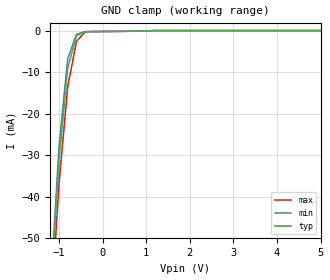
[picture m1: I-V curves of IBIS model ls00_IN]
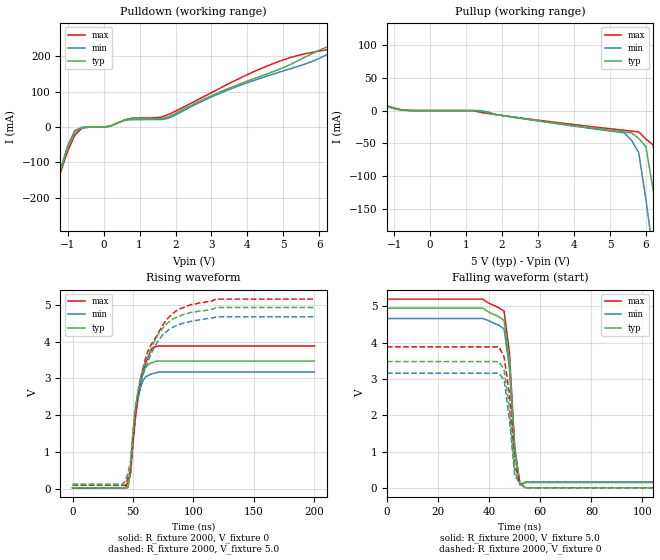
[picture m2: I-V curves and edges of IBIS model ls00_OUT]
|   TEXAS INSTRUMENTS INCORPORATED
|   Standard Linear and Logic Group
|   IBIS Model of SN74LS00
|   QUADRUPLE 2-INPUT POSITIVE-NAND GATES
|   SOIC 14-pin (D), SOP 14-pin (NS), SSOP 14-pin (DB), P-DIP 14-pin (N)
[IBIS Ver]   3.2
[Comment Char]  |_char
[File Name]   sn74ls00.ibs
[File Rev]   3.2
|[Date]   11/11/04
[Source]   File originated at Texas Instruments, Inc.
[Notes]   The following is a sample IBIS file for the LS00.
   - FILE REV HISTORY
   - 3.2 Re-Release IBIS file on 11/11/04
   - Power clamp data deleted as there is no power-clamp diode.
   - All test data contained in this file are derived from
   actual measurements.
   - The measurement used NS package.
   - File created by Nobuhisa Ohtsubo, SLL Product Engineering.
[Disclaimer] Property of Texas Instruments Incorporated.  Unauthorized
   reproduction and/or distribution is strictly prohibited.
   This product is protected under copyright law.
   Created 2000, (C) Copyright 2000, Texas Instruments Inc.,
   All Rights Reserved.
   UNLESS THERE IS A SIGNED, WRITTEN AGREEMENT TO THE
   CONTRARY, TEXAS INSTRUMENTS () IS PROVIDING THE IBIS
   MODELS  AND WITHOUT ANY WARRANTY, EXPRESSED OR
   IMPLIED.  TI assumes no liability for:
   1) the accuracy of the IBIS models provided to your
   company;
   2) the proper functioning of these IBIS Models in your
   design or for any resulting applications; or
   3) infringement of patents, copyrights or intellectual
   property rights resulting from your use of these IBIS
   models.
   TI provides IBIS Models as a service to our customers.
   You and your company shall not distribute, sell or give
   these models to anyone else without prior written
   permission from TI.
   TI reserves the right to make changes to our products or
   to discontinue any semiconductor product or service
   without notice, and advises our customers to obtain the
   latest version of relevant information to verify, before
   placing orders, that the information being relied on is
   current.
   Please be aware that your receipt and use of the IBIS
   information provided shall serve as acceptance of these
   terms and conditions.  If you do not accept these terms,
   you should return or destroy the IBIS models and any
   other accompanying information immediately.
|   Component ls00_D
[Component]   ls00_D
[Manufacturer]  Texas Instruments, Inc.
[Package]
|   typ   min   max
R_pkg   0.031   0.028   0.034
L_pkg   3.109nH   2.462nH   3.889nH
C_pkg   0.473pF   0.363pF   0.628pF
[Pin]   signal_name   model_name   R_pin   L_pin   C_pin
1   1A   ls00_IN   0.033   3.854nH   0.622pF
2   1B   ls00_IN   0.032   3.188nH   0.473pF
3   1Y   ls00_OUT   0.028   2.462nH   0.377pF
4   2A   ls00_IN   0.031   2.596nH   0.363pF
5   2B   ls00_IN   0.028   2.521nH   0.372pF
6   2Y   ls00_OUT   0.034   3.250nH   0.476pF
7   GND   GND   0.034   3.889nH   0.628pF
8   3Y   ls00_OUT   0.034   3.889nH   0.628pF
9   3A   ls00_IN   0.034   3.250nH   0.476pF
10   3B   ls00_IN   0.028   2.521nH   0.372pF
11   4Y   ls00_OUT   0.031   2.596nH   0.364pF
12   4A   ls00_IN   0.028   2.462nH   0.377pF
13   4B   ls00_IN   0.032   3.188nH   0.473pF
14   VCC   POWER   0.033   3.854nH   0.622pF
|   Component ls00_NS
[Component]   ls00_NS
[Manufacturer]  Texas Instruments, Inc.
[Package]
|   typ   min   max
R_pkg   0.045   0.039   0.054
L_pkg   3.796nH   2.561nH   4.952nH
C_pkg   0.528pF   0.288pF   0.710pF
[Pin]   signal_name   model_name   R_pin   L_pin   C_pin
1   1A   ls00_IN   0.047   4.867nH   0.706pF
2   1B   ls00_IN   0.051   4.083nH   0.592pF
3   1Y   ls00_OUT   0.041   2.915nH   0.376pF
4   2A   ls00_IN   0.039   2.561nH   0.288pF
5   2B   ls00_IN   0.041   3.101nH   0.430pF
6   2Y   ls00_OUT   0.047   4.047nH   0.589pF
7   GND   GND   0.051   4.909nH   0.700pF
8   3Y   ls00_OUT   0.045   4.784nH   0.694pF
9   3A   ls00_IN   0.054   4.176nH   0.597pF
10   3B   ls00_IN   0.039   3.287nH   0.449pF
11   4Y   ls00_OUT   0.039   2.586nH   0.294pF
12   4A   ls00_IN   0.040   2.802nH   0.371pF
13   4B   ls00_IN   0.049   4.080nH   0.593pF
14   VCC   POWER   0.052   4.952nH   0.710pF
|   Component ls00_DB
[Component]   ls00_DB
[Manufacturer]  Texas Instruments, Inc.
[Package]
|   typ   min   max
R_pkg   0.044   0.041   0.046
L_pkg   3.551nH   3.258nH   3.927nH
C_pkg   0.402pF   0.360pF   0.421pF
[Pin]   signal_name   model_name   R_pin   L_pin   C_pin
1   1A   ls00_IN   0.046   3.927nH   0.408pF
2   1B   ls00_IN   0.044   3.587nH   0.421pF
3   1Y   ls00_OUT   0.041   3.289nH   0.398pF
4   2A   ls00_IN   0.042   3.258nH   0.360pF
5   2B   ls00_IN   0.041   3.286nH   0.403pF
6   2Y   ls00_OUT   0.044   3.586nH   0.421pF
7   GND   GND   0.046   3.927nH   0.408pF
8   3Y   ls00_OUT   0.046   3.927nH   0.408pF
9   3A   ls00_IN   0.044   3.586nH   0.421pF
10   3B   ls00_IN   0.041   3.286nH   0.403pF
11   4Y   ls00_OUT   0.043   3.258nH   0.360pF
12   4A   ls00_IN   0.041   3.289nH   0.398pF
13   4B   ls00_IN   0.044   3.587nH   0.421pF
14   VCC   POWER   0.046   3.927nH   0.408pF
|   Component ls00_N
[Component]   ls00_N
[Manufacturer]   Texas Instruments, Inc.
[Package]
|   typ   min   max
R_pkg   4.500e-02   3.700e-02   6.300e-02
L_pkg   5.407e-09   3.922e-09   6.942e-09
C_pkg   3.890e-13   2.050e-13   6.040e-13
[Pin]   signal_name   model_name   R_pin   L_pin   C_pin
1   1A   ls00_IN   6.300e-02   6.942e-09   6.040e-13
2   1B   ls00_OUT   3.700e-02   6.200e-09   4.060e-13
3   1Y   ls00_IN   4.200e-02   4.389e-09   3.220e-13
4   2A   ls00_OUT   3.800e-02   3.922e-09   2.050e-13
5   2B   ls00_IN   3.900e-02   4.301e-09   2.980e-13
6   2Y   ls00_OUT   3.800e-02   5.329e-09   3.560e-13
7   GND   GND   5.300e-02   6.510e-09   5.440e-13
8   3Y   ls00_OUT   5.300e-02   6.437e-09   5.390e-13
9   3A   ls00_IN   3.900e-02   5.352e-09   3.470e-13
10   3B   ls00_OUT   4.200e-02   4.473e-09   2.970e-13
11   4Y   ls00_IN   4.400e-02   4.326e-09   2.250e-13
12   4A   ls00_OUT   4.200e-02   4.295e-09   2.800e-13
13   4B   ls00_IN   4.200e-02   6.318e-09   4.180e-13
14   VCC   POWER   6.100e-02   6.900e-09   6.030e-13
| Models and submodels in the file (2): ls00_IN (Input), ls00_OUT (Output)
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|   Model ls00_IN
[Model]   ls00_IN
Model_type  Input
Polarity   Inverting
Vinl = 0.8
Vinh = 2.0
| variable   typ   min   max
C_comp   1.33pf   1.00pf   1.66pf
[Temperature Range]   25   0   70
[Voltage Range]   5.0   4.75   5.25
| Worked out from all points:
|   GND clamp passes 1 mA (typ) near -0.55 V on its own axis
[GND Clamp]
|   Voltage   I(typ)   I(min)   I(max)
-5V       -1.018A    -1.077A    -921.2mA
-1.2V     -66.4mA    -63.52mA   -70.37mA
-1V       -31.36mA   -27.9mA    -37.06mA
-800mV    -9.019mA   -6.772mA   -13.61mA
-600mV    -1.272mA   -876.1uA   -2.626mA
-400mV    -255.9uA   -254.9uA   -323.7uA
-200mV    -235.6uA   -242.4uA   -213.5uA
1.2V      -728.9nA   -2.758uA   -68.03nA
5V        8.6nA      8.752nA    16.82nA
|   Model ls00_OUT
[Model]   ls00_OUT
Model_type  Output
Polarity   Non-Inverting
Vmeas = 1.3v
Cref = 15pf
Rref = 2000
Vref = 0V
| variable   typ   min   max
C_comp   5.8pf   4.35pf   7.25pf
[Temperature Range]   25   0   70
[Voltage Range]   5.0   4.75   5.25
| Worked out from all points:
|   slope of the pulldown table from 0 to 0.75 V, typ, clamps not added: 32.8 ohm
|   slope of the pullup table from 0 to 0.75 V, typ, clamps not added: 31.9 kohm
|   rising waveform, R_fixture 2000, V_fixture 0: 20-80 % time 7.12ns typ, 6.53ns min, 8.96ns max; typ from 0.022 V to 3.47 V
|   falling waveform, R_fixture 2000, V_fixture 5.0: 20-80 % time 2.91ns typ, 2.91ns min, 2.89ns max; typ from 4.95 V to 0.156 V
|   rising waveform, R_fixture 2000, V_fixture 5.0: 20-80 % time 18.3ns typ, 17.6ns min, 19.9ns max; typ from 0.11 V to 4.93 V
|   falling waveform, R_fixture 2000, V_fixture 0: 20-80 % time 2.93ns typ, 2.92ns min, 3.01ns max; typ from 3.48 V to 0.011 V
[Pulldown]
|   Voltage   I(typ)   I(min)   I(max)
-5V       -1.623A    -1.707A    -1.473A
-1.8V     -355.8mA   -364.5mA   -338.6mA
-1.6V     -276.6mA   -280.8mA   -267.5mA
-1.2V     -124mA     -120.4mA   -129.6mA
-1V       -58.61mA   -53.03mA   -68.64mA
-800mV    -14.32mA   -10.47mA   -22.99mA
-600mV    -1.475mA   -1.096mA   -3.152mA
1.8V      28.53mA    24.12mA    35.15mA
5V        167.6mA    158.3mA    189.4mA
6.4V      233.2mA    215.8mA    221.3mA
7.8V      258.5mA    282.1mA    240.2mA
10V       292.8mA    378mA      268.4mA
[Pullup]
|   Voltage   II(typ)   I(min)   I(max)
-5V       116.3mA    125.9mA    104.1mA
-2V       26.57mA    26.24mA    26.21mA
-1V       3.179mA    2.827mA    3.873mA
1.4V      -267.2uA   -169uA     -2.666mA
5.4V      -32.59mA   -33.92mA   -30.06mA
5.6V      -33.94mA   -45.18mA   -31.27mA
5.8V      -42.24mA   -64.1mA    -32.52mA
6V        -54.87mA   -135.2mA   -43.33mA
6.2V      -120.2mA   -216.1mA   -52.23mA
6.4V      -195.4mA   -300.8mA   -110.4mA
6.6V      -275.3mA   -387.9mA   -176.9mA
10V       -1.681A    -1.881A    -1.43A
[Ramp]
| variable   typ   min   max
dV/dt_r  1.962E+00/5.182E-09  1.770E+00/4.449E-09  2.202E+00/6.445E-09
dV/dt_f  2.826E+00/2.251E-09  2.676E+00/2.415E-09  2.994E+00/2.132E-09
R_load = 2000
[Rising Waveform]
R_fixture = 2000
V_fixture = 0
V_fixture_min = 0
V_fixture_max = 0
C_fixture = 0pf
L_fixture = 0nH
|   Time   V(typ)   V(min)   V(max)
0s        21.98mV    23.41mV    20.04mV
43.75ns   22.44mV    24.19mV    20.18mV
45.83ns   32.5mV     26.19mV    189.7mV
47.92ns   507.3mV    483.6mV    378.3mV
50ns      1.494V     1.469V     1.233V
52.08ns   2.151V     2.099V     1.945V
56.25ns   2.906V     2.754V     2.858V
60.42ns   3.302V     3.047V     3.419V
66.67ns   3.437V     3.136V     3.844V
200ns     3.474V     3.176V     3.883V
[Falling Waveform]
R_fixture = 2000
V_fixture = 5.0
V_fixture_min = 4.75
V_fixture_max = 5.25
C_fixture = 0pf
L_fixture = 0nH
|   Time   V(typ)   V(min)   V(max)
0s        4.951V     4.666V     5.198V
37.5ns    4.951V     4.666V     5.198V
39.58ns   4.853V     4.612V     5.096V
43.75ns   4.717V     4.481V     4.963V
45.83ns   4.612V     4.377V     4.868V
47.92ns   3.541V     3.309V     3.73V
50ns      1.058V     992.8mV    1.131V
52.08ns   83.54mV    86.14mV    108.1mV
54.17ns   156mV      172.4mV    166.7mV
200ns     156mV      172.4mV    166.7mV
[Rising Waveform]
R_fixture = 2000
V_fixture = 5.0
V_fixture_min = 4.75
V_fixture_max = 5.25
C_fixture = 0pf
L_fixture = 0nH
|   Time   V(typ)   V(min)   V(max)
0s        110.1mV    116.9mV    89mV
43.75ns   223.4mV    228.2mV    89.85mV
47.92ns   676.2mV    731.1mV    483.5mV
52.08ns   2.26V      2.217V     2.067V
56.25ns   3.031V     2.886V     2.983V
60.42ns   3.471V     3.287V     3.557V
72.92ns   4.296V     4.122V     4.358V
85.42ns   4.659V     4.433V     4.834V
118.8ns   4.931V     4.679V     5.16V
200ns     4.931V     4.679V     5.16V
[Falling Waveform]
R_fixture = 2000
V_fixture = 0
V_fixture_min = 0
V_fixture_max = 0
C_fixture = 0pf
L_fixture = 0nH
|   Time   V(typ)   V(min)   V(max)
0s        3.482V     3.165V     3.889V
43.75ns   3.482V     3.165V     3.889V
45.83ns   3.265V     2.978V     3.609V
47.92ns   2.207V     1.891V     2.605V
50ns      451.3mV    348.9mV    663.8mV
52.08ns   125.5mV    120.8mV    139.2mV
54.17ns   12.31mV    12.58mV    14.21mV
56.25ns   11.04mV    12.44mV    13.22mV
200ns     11.04mV    12.44mV    13.22mV
